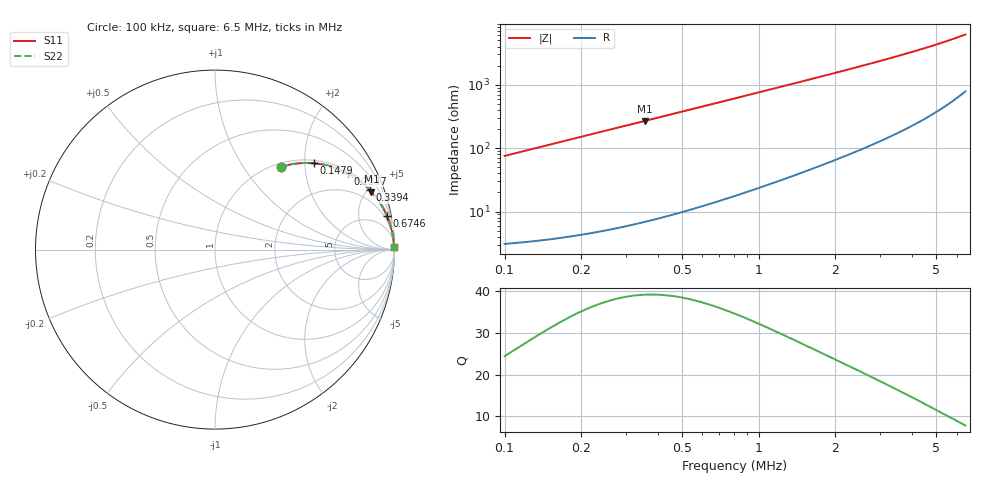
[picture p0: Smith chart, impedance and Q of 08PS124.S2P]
! Coilcraft 0805PS-124 Power Chip Inductor
! 5 February 2003
# MHZ S MA R 50
!Freq  MagS11  AngS11  MagS21  AngS21  MagS12  AngS12  MagS22  AngS22
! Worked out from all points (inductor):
!   403 points, 100 kHz to 6.5 MHz, reference 50 ohm
!   read as one part in series: L = 120 uH near 131.9 kHz
!   highest Q = 39 at 355.4 kHz (marker M1), where L = 120 uH
!   S11 on the Smith chart (normalised r, x): 100 kHz: 1.06, +1.51; 147.9 kHz: 1.07, +2.23; 227.7 kHz: 1.09, +3.43; 339.4 kHz: 1.13, +5.12; 674.6 kHz: 1, +10; 6.5 MHz: open
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0.1  0.5908 51.5  0.783 -36.2  0.783 -36.2  0.5908 51.5
0.11596  0.6467 47.6  0.7391 -40.3  0.7391 -40.3  0.6467 47.6
0.14788  0.7329 41.0  0.657 -47.1  0.657 -47.1  0.7329 41.0
0.1798  0.7937 35.8  0.5852 -52.5  0.5852 -52.5  0.7937 35.8
0.22768  0.8541 29.8  0.4973 -58.6  0.4973 -58.6  0.8541 29.8
0.27556  0.8921 25.4  0.4291 -63.1  0.4291 -63.1  0.8921 25.4
0.3394  0.9235 21.1  0.3606 -67.4  0.3606 -67.4  0.9235 21.1
0.35536  0.9292 20.3  0.3466 -68.3  0.3466 -68.3  0.9292 20.3
0.4192  0.9466 17.4  0.2992 -71.1  0.2992 -71.1  0.9466 17.4
0.48304  0.9581 15.2  0.2627 -73.3  0.2627 -73.3  0.9581 15.2
0.5788  0.9692 12.8  0.2217 -75.7  0.2217 -75.7  0.9692 12.8
0.67456  0.9762 11.0  0.1915 -77.4  0.1915 -77.4  0.9762 11.0
0.898  0.9851 8.3  0.1449 -80.0  0.1449 -80.0  0.9851 8.3
1.16932  0.9901 6.4  0.1115 -81.7  0.1115 -81.7  0.9901 6.4
1.39276  0.9923 5.4  0.09358 -82.6  0.09358 -82.6  0.9923 5.4
1.64812  0.9939 4.5  0.07889 -83.3  0.07889 -83.3  0.9939 4.5
2.23864  0.9958 3.3  0.05751 -84.1  0.05751 -84.1  0.9958 3.3
2.7334  0.9966 2.7  0.04653 -84.4  0.04653 -84.4  0.9966 2.7
3.30796  0.9971 2.2  0.03777 -84.5  0.03777 -84.5  0.9971 2.2
4.37728  0.9976 1.6  0.02731 -84.2  0.02731 -84.2  0.9976 1.6
5.4466  0.9978 1.2  0.02068 -83.3  0.02068 -83.3  0.9978 1.2
6.5  0.9978 0.9  0.01609 -81.8  0.01609 -81.8  0.9978 0.9
